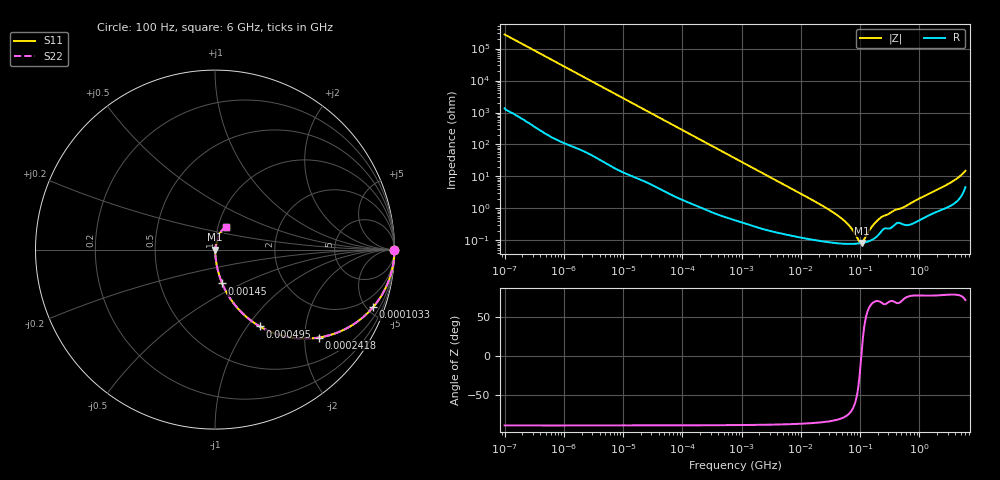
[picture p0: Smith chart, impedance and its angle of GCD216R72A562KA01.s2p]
!Murata Part Number: GCD216R72A562KA01
!These Parameters are Measured in Series Mode Connection
!Data Generated on Jan 08, 2026
!  o--ll--o
!Port1  Port2
!  o------o
!Operation Temp=25[degC], DC Bias Voltage=0[V]
!Freq. Start=100[Hz] Stop=6[GHz] 401[Steps]
# Hz S RI R 50
!Freq.(Hz) S11(Real) S11(Imag) S21(Real) S21(Imag) S12(Real) S12(Imag) S22(Real) S22(Imag)
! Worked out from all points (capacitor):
!   401 points, 100 Hz to 6 GHz, reference 50 ohm
!   read as one part in series: C = 5.75 nF near 109 Hz
!   lowest |Z| = 83.2 mohm at 106.7 MHz (marker M1)
!   series resonance near 105 MHz, so ESL is about 400 pH
!   S11 on the Smith chart (normalised r, x): 100 Hz: open; 103.3 kHz: 1.04, -5.46; 241.8 kHz: 1.02, -2.34; 495 kHz: 1.01, -1.15; 1.45 MHz: 1.01, -0.39; 6 GHz: 1.09, +0.29
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100  1 -0.000362  1.9e-06 0.000362  1.9e-06 0.000362  1 -0.000362
2008  0.9999 -0.00721  8.61e-05 0.00721  8.61e-05 0.00721  0.9999 -0.00721
12592  0.9978 -0.0449  0.00224 0.0449  0.00224 0.0449  0.9978 -0.0449
40335  0.979 -0.1403  0.021 0.1403  0.021 0.1403  0.979 -0.1403
103284  0.8802 -0.3214  0.1198 0.3214  0.1198 0.3214  0.8802 -0.3214
241822  0.5776 -0.49  0.4224 0.49  0.4224 0.49  0.5776 -0.49
495019  0.2498 -0.4281  0.7502 0.4281  0.7502 0.4281  0.2498 -0.4281
774597  0.1219 -0.3214  0.8781 0.3214  0.8781 0.3214  0.1219 -0.3214
1449809  0.04 -0.1887  0.96 0.1887  0.96 0.1887  0.04 -0.1887
3882480  0.0072 -0.0734  0.9928 0.0734  0.9928 0.0734  0.0072 -0.0734
1.555665e7  0.00139 -0.0184  0.9986 0.0184  0.9986 0.0184  0.00139 -0.0184
5.211241e7  0.000805 -0.00432  0.9992 0.00432  0.9992 0.00432  0.000805 -0.00432
7.129496e7  0.000782 -0.00227  0.9992 0.00227  0.9992 0.00227  0.000782 -0.00227
9.753859e7  0.000807 -0.000425  0.9992 0.000425  0.9992 0.000425  0.000807 -0.000425
1.066761e8  0.000826 9.11e-05  0.9992 -9.11e-05  0.9992 -9.11e-05  0.000826 9.11e-05
1.166697e8  0.000853 0.000611  0.9991 -0.000611  0.9991 -0.000611  0.000853 0.000611
1.526266e8  0.001 0.00224  0.999 -0.00224  0.999 -0.00224  0.001 0.00224
1.909225e8  0.00132 0.00376  0.9987 -0.00376  0.9987 -0.00376  0.00132 0.00376
2.283698e8  0.00193 0.00496  0.9981 -0.00496  0.9981 -0.00496  0.00193 0.00496
3.124326e8  0.00239 0.00652  0.9976 -0.00652  0.9976 -0.00652  0.00239 0.00652
2.931063e9  0.0134 0.053  0.9866 -0.053  0.9866 -0.053  0.0134 0.053
6e9  0.0618 0.1284  0.9382 -0.1284  0.9382 -0.1284  0.0618 0.1284
